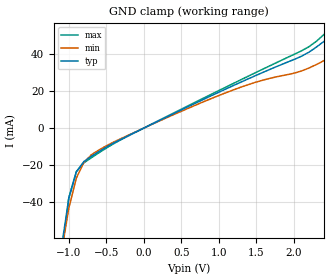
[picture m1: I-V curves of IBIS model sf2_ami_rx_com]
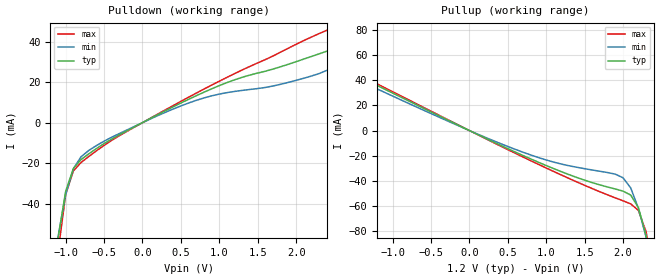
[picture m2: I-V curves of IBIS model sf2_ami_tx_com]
|   Microsemi Corporation
|   SmarFusion2/IGLOO2 Commercial IBIS-AMI Models
[IBIS ver]   5.0
[File name]   sf2_igl2_ami_com.ibs
[File Rev]   1.3
[Date]   February 1, 2019
[Disclaimer] These IBIS Models are Provided "As is" with NO WARRANTY
   whatsoever and signal integrity software specifically disclaims any
   implied warranties of merchantability, fitness for a particular
   purpose or against infringement.
[Source]   Original model developed in collaboration with Sigrity. Optimized by SiSoft.
[Notes]   Known limitations: Main tap is limited to maximum amplitude setting only
   and cannot be adjusted.
-Revision History:
1.4: February 1, 2019
   * Added model limitation note on abicdr_tx.ami and sf2_igl2_ami_com.ibs files.
1.3: July 22, 2015
   * Added Algorithmic Model to support 64-bit Window environment
1.2: April 2, 2015
   * Added new RLC packages in Package section.
1.1: June 12, 2014
   * Updated Package section.
   * Consolidated the IGLOO2 and SmartFusion2 IBIS AMI Model
   * Updated the RX .ami model to clarify comments.
1.05: 6 November 2013
   Based on the model 1.0 model supplied by Microsemi dated 18 March 2013.
   This model has been optimized for use with SiSoft's QCD Simulator. Points of note:
   * Updated [Ramp] data to correct single-ended / differential issues
   * Updated C_comp values using data provided by Microsemi
   * Updated TX .ami file to disable auto EQ mode (does not work with QCD)
   * Included TX jitter data derived from PCIe Gen2 compliance testing
   * Signed models as QCD Certified
1.0: 18 March 2013 20:52:13
   * Original model supplied by Microsemi
[Copyright]  (c) 2014, Microsemi Corporation, All Rights Reserved.
[Component]  SF2_IGL2_ibis_ami_com
[Manufacturer] Microsemi Corporation
[Package]
|   typ   min   max
| M2S/M2GL005
|R_pkg   0.72029   0.51528   1.0002   |005-FG484
|L_pkg   5.797e-9   4.155e-9   8.073e-9   |005-FG484
|C_pkg   1.116e-12   7.907e-13   1.753e-12   |005-FG484
|R_pkg   0.27009   0.041405   0.45769   |005-VF256
|L_pkg   4.091e-9   8.144e-10   7.139e-9   |005-VF256
|C_pkg   9.403e-13   6.174e-13   2.852e-12   |005-VF256
|R_pkg   0.47234   0.051444   0.70881   |005-VF400
|L_pkg   3.73e-9   4.383e-10   5.254e-9   |005-VF400
|C_pkg   9.092e-13   5.433e-13   3.219e-12   |005-VF400
|R_pkg   0.45289   0.15933   0.53232   |005-TQ144
|L_pkg   7.371e-9   3.475e-9   8.58e-9   |005-TQ144
|C_pkg   5.58e-13   4.777e-13   2.009e-12   |005-TQ144
| M2S/M2GL010
|R_pkg   0.66635   0.053835   1.0211   |010-FG484
|L_pkg   5.248e-9   6.178e-10   7.432e-9   |010-FG484
|C_pkg   1.306e-12   8.624e-13   3.748e-12   |010-FG484
|R_pkg   0.45429   0.057027   0.75756   |010-VF256
|L_pkg   3.996e-9   5.786e-10   5.727e-9   |010-VF256
|C_pkg   7.828e-13   3.988e-13   2.733e-12   |010-VF256
|R_pkg   0.42093   0.053275   0.67244   |010-VF400
|L_pkg   3.621e-9   5.054e-10   5.523e-9   |010-VF400
|C_pkg   1.012e-12   7.358e-13   4.005e-12   |010-VF400
|R_pkg   1.0678   0.95825   1.2776   |010-TQ144
|L_pkg   6.828e-9   5.979e-9   8.176e-9   |010-TQ144
|C_pkg   5.261e-13   4.459e-13   6.909e-13   |010-TQ144
| M2S/M2GL025
|R_pkg   0.62161   0.045855   0.88864   |025-FG484
|L_pkg   4.896e-9   4.955e-10   6.635e-9   |025-FG484
|C_pkg   1.283e-12   7.336e-13   4.781e-12   |025-FG484
|R_pkg   0.5113   0.081888   0.79004   |025-VF256
|L_pkg   4.3e-9   8.149e-10   6.356e-9   |025-VF256
|C_pkg   9.84e-13   5.422e-13   3.998e-12   |025-VF256
|R_pkg   0.56911   0.07806   0.87745   |025-VF400
|L_pkg   4.165e-9   7.124e-10   5.915e-9   |025-VF400
|C_pkg   1.037e-12   6.508e-13   4.436e-12   |025-VF400
|R_pkg   0.98263   0.44871   1.4996   |025-FCS325
|L_pkg   2.992e-9   1.127e-9   4.449e-9   |025-FCS325
|C_pkg   7.686e-13   4.28e-13   1.093e-12   |025-FCS325
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R_pkg   0.65025   0.050477   0.98075   |050-FG896
L_pkg   8.654e-9   4.198e-9   1.391e-8   |050-FG896
C_pkg   1.881e-12   1.117e-12   7.153e-12   |050-FG896
|R_pkg   0.64708   0.10714   1.1617   |050-FG484
|L_pkg   4.885e-9   8.618e-10   8.001e-9   |050-FG484
|C_pkg   1.224e-12   7.009e-13   2.089e-12   |050-FG484
|R_pkg   0.51212   0.082442   0.77494   |050-VF400
|L_pkg   3.938e-9   7.719e-10   5.981e-9   |050-VF400
|C_pkg   9.187e-13   5.253e-13   3.26e-12   |050-VF400
|R_pkg   0.87592   0.4729   1.2989   |050-FCS325
|L_pkg   2.542e-9   1.291e-9   3.732e-9   |050-FCS325
|C_pkg   6.621e-13   4.118e-13   9.479e-13   |050-FCS325
| M2S/M2GL060
|R_pkg   0.58359   0.09068   0.74939   |060-FG676
|L_pkg   5.269e-9   9e-10   6.659e-9   |060-FG676
|C_pkg   1.37e-12   5.634e-13   4.553e-12   |060-FG676
|R_pkg   0.56892   0.053004   0.79188   |060-FG484
|L_pkg   4.842e-9   5.148e-10   6.754e-9   |060-FG484
|C_pkg   1.575e-12   9.705e-13   7.459e-12   |060-FG484
|R_pkg   0.52053   0.072609   0.81109   |060-VF400
|L_pkg   4.301e-9   6.587e-10   6.035e-9   |060-VF400
|C_pkg   7.921e-13   3.769e-13   2.744e-12   |060-VF400
|R_pkg   0.8976   0.13778   1.274   |060-FCS325
|L_pkg   2.041e-9   3.18e-10   3.117e-9   |060-FCS325
|C_pkg   8.765e-13   4.713e-13   3.781e-12   |060-FCS325
| M2S/M2GL090
|R_pkg   0.63738   0.081807   0.76878   |090-FG676
|L_pkg   4.82e-9   7.761e-10   6.16e-9   |090-FG676
|C_pkg   1.49e-12   1.064e-12   7.809e-12   |090-FG676
|R_pkg   0.64363   0.064239   0.93501   |090-FG484
|L_pkg   4.937e-9   6.079e-10   6.828e-9   |090-FG484
|C_pkg   1.588e-12   6.307e-13   1.263e-11   |090-FG484
|R_pkg   0.82801   0.25425   1.2469   |090-FCS325
|L_pkg   2.074e-9   7.125e-10   3.565e-9   |090-FCS325
|C_pkg   9.158e-13   3.94e-13   1.405e-12   |090-FCS325
| M2S/M2GL150
|R_pkg   0.67258   0.11704   1.2705   |150-FCV484
|L_pkg   3.013e-9   9.675e-10   4.881e-9   |150-FCV484
|C_pkg   1.45e-12   7.195e-13   2.327e-12   |150-FCV484
|R_pkg   0.46246   0.10876   0.7535   |150-FCS536
|L_pkg   1.775e-9   4.138e-10   2.986e-9   |150-FCS536
|C_pkg   9.306e-13   4.484e-13   5.765e-12   |150-FCS536
|R_pkg   0.86225   0.11212   1.7907   |150-FC1152
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[Pin]   signal_name   model_name   R_pin  L_pin  C_pin
1p   sf2_tx_p   sf2_ami_tx_com   NA   NA   NA
1n   sf2_tx_n   sf2_ami_tx_com   NA   NA   NA
2p   sf2_rx_p   sf2_ami_rx_com   NA   NA   NA
2n   sf2_rx_n   sf2_ami_rx_com   NA   NA   NA
[Diff_Pin] inv_pin vdiff tdelay_typ tdelay_min tdelay_max
1p   1n   0.1V  NA   NA   NA
2p   2n   0.1V  NA   NA   NA
| Models and submodels in the file (2): sf2_ami_rx_com (Input), sf2_ami_tx_com (Output)
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|   Model sf2_ami_rx_com
[Model] sf2_ami_rx_com
|SiSoft ModelSignature1 dd25d4250606c5a9568d9513a163a207e57de67c17f73abc8b005ecaca24aea6 Certified
Model_type Input
C_comp 0.914p 0.471p 1.37p
Vinh = 0.55
Vinl = 0.45
| Differential package model for post-route analysis
|SiSoft Diff_Package SF2_FG896_472673AP0A_0308_PCIE2_TxRx.s4p.smod s_SF2_FG896_472673AP0A_0308_PCIE2_TxRx
[Algorithmic Model]
Executable Windows_VisualStudio7.1.3088_32 abicdr_rx.dll   abicdr_rx.ami
Executable Windows_VisualStudio7.1.3088_64 abicdr_x64_rx.dll  abicdr_rx.ami
Executable Linux_gcc3.2.3_64   abicdr_rh64_rx.dll abicdr_rx.ami
[End Algorithmic Model]
[Temperature Range]   25C   85C   0C
[Voltage Range]   1.2V   1.14V  1.26V
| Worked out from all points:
|   GND clamp passes 1 mA (typ) near -0.05 V on its own axis
[GND Clamp]
|Voltage   I(typ)   I(min)   I(max)
-2.5V     -710.8mA   -586.4mA   -913.9mA
-1.1V     -65.27mA   -68.16mA   -70.07mA
-1V       -38.09mA   -43.46mA   -37.77mA
-900mV    -23.87mA   -27.21mA   -23.61mA
-800mV    -18.2mA    -18.66mA   -18.9mA
-700mV    -15.32mA   -14.5mA    -16.1mA
-300mV    -5.977mA   -5.605mA   -6.214mA
1V        19.46mA    17.68mA    20.37mA
1.5V      28.68mA    24.99mA    30.3mA
2.1V      38.95mA    30.97mA    41.89mA
2.3V      43.94mA    34.49mA    47.08mA
2.5V      50.17mA    38.74mA    54.71mA
|   Model sf2_ami_tx_com
[Model] sf2_ami_tx_com
|SiSoft ModelSignature1 95aea496e6c87737188cb2b58ec32bbeb15ff6f85179c3186e5c97671b8de29c Certified
Model_type Output
C_comp 0.914p 0.471p 1.37p
Cref = 0
Vref = 0.5
Rref = 50
Vmeas = 0.6
| Differential package model for post-route analysis
|SiSoft Diff_Package SF2_FG896_472673AP0A_0308_PCIE2_TxRx.s4p.smod s_SF2_FG896_472673AP0A_0308_PCIE2_TxRx
[Algorithmic Model]
Executable Windows_VisualStudio7.1.3088_32 abicdr_tx.dll   abicdr_tx.ami
Executable Windows_VisualStudio7.1.3088_64 abicdr_x64_tx.dll  abicdr_tx.ami
Executable Linux_gcc3.2.3_64   abicdr_rh64_tx.dll abicdr_tx.ami
[End Algorithmic Model]
[Temperature Range]   25C   85C   0C
[Voltage Range]   1.2V   1.14V   1.26V
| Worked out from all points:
|   slope of the pulldown table from 0 to 0.18 V, typ, clamps not added: 50.4 ohm
|   slope of the pullup table from 0 to 0.18 V, typ, clamps not added: 34.2 ohm
[Pulldown]
|Voltage   I(typ)   I(min)   I(max)
-2.5V     -663.6mA   -536.5mA   -868.1mA
-1.1V     -57.52mA   -56.53mA   -64.41mA
-1V       -33.95mA   -35.57mA   -35.56mA
-900mV    -22.69mA   -22.79mA   -23.9mA
-800mV    -18.27mA   -16.87mA   -19.7mA
-600mV    -12.82mA   -11.35mA   -13.94mA
100mV     1.995mA    1.764mA    2.136mA
700mV     13.31mA    11.02mA    14.59mA
1.2V      21.19mA    15.44mA    24.26mA
1.8V      27.64mA    18.98mA    34.89mA
2.3V      34.02mA    24.28mA    44.02mA
2.5V      36.63mA    27.73mA    47.25mA
[Pullup]
|Voltage   I(typ)   I(min)   I(max)
-3.7V     173.4mA    158.8mA    198.1mA
-2.7V     88.71mA    85.75mA    92.74mA
-2.5V     78.42mA    75.59mA    81.05mA
-1.8V     54.07mA    50.5mA     55.79mA
300mV     -8.734mA   -7.767mA   -9.169mA
1.1V      -30.38mA   -25.18mA   -32.67mA
1.9V      -46.55mA   -34.73mA   -53.63mA
2V        -48.22mA   -37.61mA   -55.93mA
2.1V      -51.37mA   -45.64mA   -58.41mA
2.2V      -61.31mA   -61.91mA   -63.55mA
2.3V      -83.51mA   -84.91mA   -80.51mA
3.6V      -622.5mA   -520.8mA   -788.7mA
[Ramp]
| variable   typ   min   max
dV/dt_r 0.3912/8.652e-11   0.3470/8.992e-11   0.4197/8.315e-11
dV/dt_f 0.3912/7.387e-11   0.3470/7.792e-11   0.4197/7.300e-11
R_load = 50
|End [Model] sf2_ami_tx_com
|End [Component]
